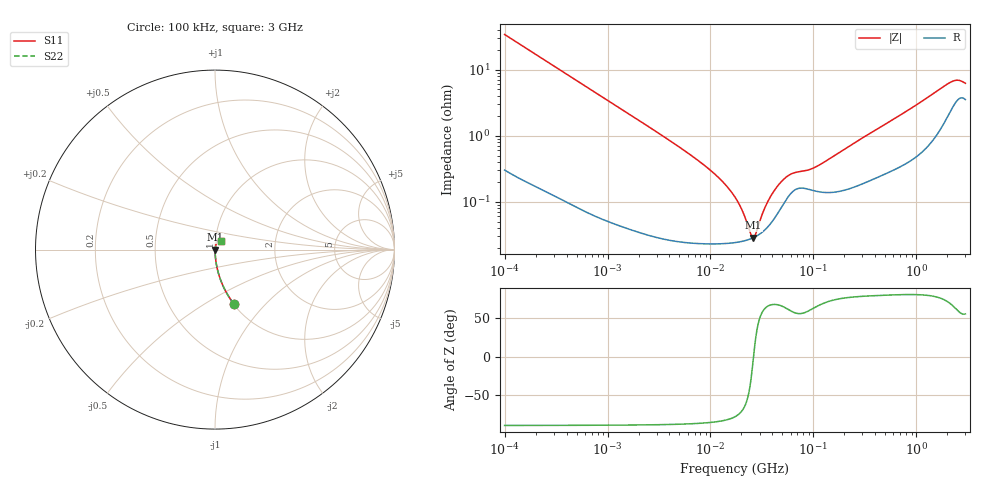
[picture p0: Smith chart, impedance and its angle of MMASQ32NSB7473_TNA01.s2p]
! MMASQ32NSB7473_TNA01  S-PARAMETER MODEL  ( Standard Model )
! Model Generated by TAIYO YUDEN Corporation (http://www.ty-top.com)
! Version 1.0
! TAIYO YUDEN Control No. 220601
! Copyright(c) 2013 TAIYO YUDEN CO.,LTD. All Rights Reserved.
! Product Description (link to TY-COMPAS)
! https://ds.yuden.co.jp/TYCOMPAS/or/detail?pn=MMASQ32NSB7473KTNA01&u=M
! Products Name : Multilayer Ceramic Capacitors
! Characteristics :
!  Capacitance : 0.047 [uF] , Rated Voltage : 250 [V] , TCC : X7R
!  Case Size : 3.2 x 2.5 / 0.126 x 0.098 [mm/inch] , Thickness : 1.9 / 0.075 [mm/inch]
!  (Conditions: Temperature = 25 [degC] , DC Bias Voltage = 0 [V])
! External Node Assignments :
!  1  o---| |---o  2
! GND o---------o GND
! Frequency Range : 100kHz  -  3GHz  [ 401 STEP ]
# MHZ S RI R 50
! Freq[MHz].  S11 Real  S11 Imag  S21 Real  S21 Imag  S12 Real  S12 Imag  S22 Real  S22 Imag
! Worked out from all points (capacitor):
!   401 points, 100 kHz to 3 GHz, reference 50 ohm
!   read as one part in series: C = 46.9 nF near 105.3 kHz
!   lowest |Z| = 28.6 mohm at 26.16 MHz (marker M1)
!   series resonance near 26.22 MHz, so ESL is about 790 pH
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0.1  0.1052 -0.3024  0.8948 0.3024  0.8948 0.3024  0.1052 -0.3024
0.228123  0.0232 -0.1455  0.9768 0.1455  0.9768 0.1455  0.0232 -0.1455
0.562235  0.00443 -0.0605  0.9956 0.0605  0.9956 0.0605  0.00443 -0.0605
3.161081  0.000398 -0.0108  0.9996 0.0108  0.9996 0.0108  0.000398 -0.0108
6.3393  0.000264 -0.00516  0.9997 0.00516  0.9997 0.00516  0.000264 -0.00516
10.08119  0.000239 -0.00295  0.9998 0.00295  0.9998 0.00295  0.000239 -0.00295
14.09348  0.000236 -0.00177  0.9998 0.00177  0.9998 0.00177  0.000236 -0.00177
17.7727  0.000243 -0.00108  0.9998 0.00108  0.9998 0.00108  0.000243 -0.00108
20.74485  0.000254 -0.000642  0.9997 0.000642  0.9997 0.000642  0.000254 -0.000642
24.84619  0.000276 -0.000148  0.9997 0.000148  0.9997 0.000148  0.000276 -0.000148
26.16047  0.000286 -6.64e-06  0.9997 6.64e-06  0.9997 6.64e-06  0.000286 -6.64e-06
27.54426  0.000298 0.000136  0.9997 -0.000136  0.9997 -0.000136  0.000298 0.000136
32.15051  0.000351 0.000574  0.9996 -0.000574  0.9996 -0.000574  0.000351 0.000574
35.64176  0.000408 0.000879  0.9996 -0.000879  0.9996 -0.000879  0.000408 0.000879
40.54368  0.000523 0.00127  0.9995 -0.00127  0.9995 -0.00127  0.000523 0.00127
47.32384  0.000758 0.00175  0.9992 -0.00175  0.9992 -0.00175  0.000758 0.00175
61.23616  0.00137 0.00226  0.9986 -0.00226  0.9986 -0.00226  0.00137 0.00226
97.38194  0.0015 0.00279  0.9985 -0.00279  0.9985 -0.00279  0.0015 0.00279
547.5153  0.00305 0.0159  0.9969 -0.0159  0.9969 -0.0159  0.00305 0.0159
2091.327  0.0244 0.0563  0.9756 -0.0563  0.9756 -0.0563  0.0244 0.0563
2504.792  0.0362 0.0558  0.9638 -0.0558  0.9638 -0.0558  0.0362 0.0558
3000  0.0362 0.0475  0.9638 -0.0475  0.9638 -0.0475  0.0362 0.0475
